FUNCTION_BLOCK FB_Generator IMPLEMENTS I_Generator
VAR_INPUT
END_VAR
VAR_OUTPUT
END_VAR
VAR
	tCycletime: TIME;
	fbTon1: TON;
	bFlashVar: BOOL;
END_VAR

{warning 'add method implementation'}
METHOD M_Flash : BOOL
fbTon1(IN:=NOT fbTon1.Q , 
	PT:=tCycletime , 
	Q=> , 
	ET=> );

IF fbTon1.Q THEN
	bFlashVar := NOT bFlashVar;
END_IF

M_Flash := bFlashVar;
END_METHOD

{warning 'add property implementation'}
PROPERTY P_Cycletime : TIME
GET
P_Cycletime:=tCycletime;
END_GET
SET
IF P_Cycletime < T#50MS THEN
	tCycletime := T#50MS;
ELSIF P_Cycletime > T#5S THEN
	tCycletime := T#5S;
ELSE
	tCycletime := P_Cycletime;
END_IF
END_SET
END_PROPERTY

{warning 'add property implementation'}
PROPERTY P_Vendor : STRING
GET
P_Vendor := 'Company X';
END_GET
END_PROPERTY

END_FUNCTION_BLOCK
